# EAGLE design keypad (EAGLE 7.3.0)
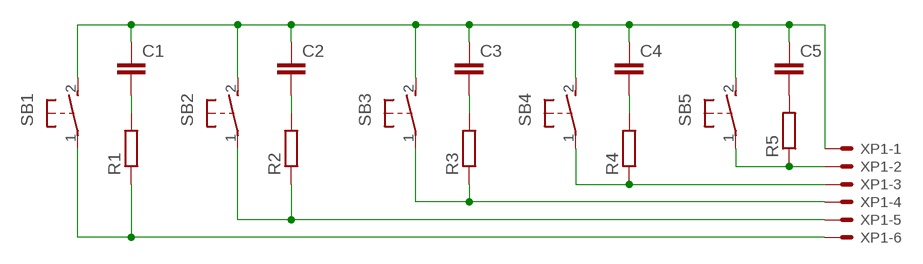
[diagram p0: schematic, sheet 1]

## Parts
C1  C-EUC0603  [C0603]
C2  C-EUC0603  [C0603]
C3  C-EUC0603  [C0603]
C4  C-EUC0603  [C0603]
C5  C-EUC0603  [C0603]
R1  R-EU_R0603  [R0603]
R2  R-EU_R0603  [R0603]
R3  R-EU_R0603  [R0603]
R4  R-EU_R0603  [R0603]
R5  R-EU_R0603  [R0603]
SB1  DTSM-3  [DTSM-3]
SB2  DTSM-3  [DTSM-3]
SB3  DTSM-3  [DTSM-3]
SB4  DTSM-3  [DTSM-3]
SB5  DTSM-3  [DTSM-3]
XP1  53398-06  [53398-06]

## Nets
COM: C1.1 C2.1 C3.1 C4.1 C5.1 SB1.2 SB2.2 SB3.2 SB4.2 SB5.2 XP1.1
DN: R4.1 SB4.1 XP1.3
ENT: R5.1 SB5.1 XP1.2
MODE: R2.1 SB2.1 XP1.5
N$1: C1.2 R1.2
N$2: C2.2 R2.2
N$3: C3.2 R3.2
N$4: C4.2 R4.2
N$5: C5.2 R5.2
ON: R1.1 SB1.1 XP1.6
UP: R3.1 SB3.1 XP1.4

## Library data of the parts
C1-C5 = resistor:C-EU: CAPACITOR, European symbol
R1-R5 = resistor:R-EU_: RESISTOR, European symbol
SB1-SB5 = switch-tact:DTSM-3
XP1 = con-molex:53?-06: CONNECTOR wire to board 1.25 mm (.049 inch) pitch header; OC_FARNELL: 1125368; OC_NEWARK: unknown

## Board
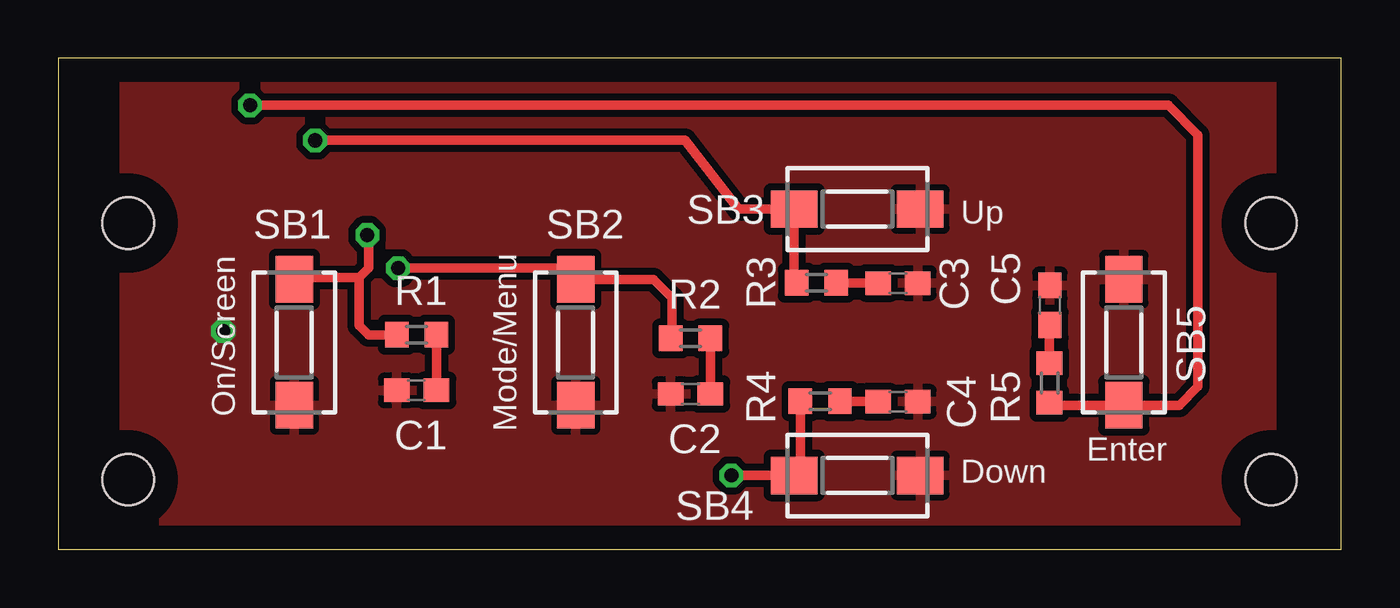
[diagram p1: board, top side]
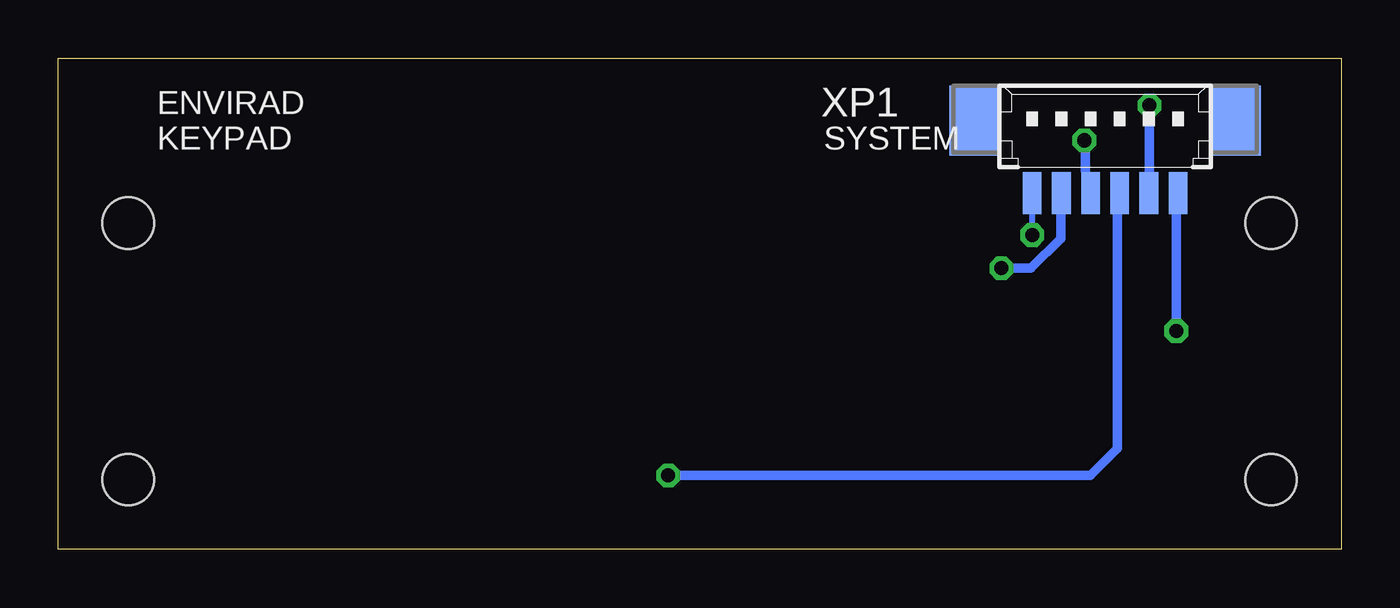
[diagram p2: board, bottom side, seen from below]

Size 55 x 21.07 mm. Coordinates in mm from the lower left corner, seen from the top.
Outline: 0,0 55,0 55,21.07 0,21.07 0,0
Copper layers (1*16): Top 0.035mm / dielectric 1.5mm / Bottom 0.035mm
Design rules "default *": minimum track width 10mil, minimum drill 20mil, track to track 8mil, track to pad 8mil, pad to pad 8mil, via to via 8mil, smd to smd 8mil, copper to edge 40mil, drill to drill 8mil, minimum pad ring 10mil, minimum via ring 8mil, stop-mask expansion 4mil, vias tented up to drill 24mil, thermal gap 10mil
Holes 2.2 mm at 3,3 52,3 52,14 3,14

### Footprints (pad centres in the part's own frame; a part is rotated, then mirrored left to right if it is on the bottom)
C0603 = smd 1.1 x 1: 1 -0.85,0; 2 0.85,0
R0603 = smd 1 x 1.1: 1 -0.85,0; 2 0.85,0
DTSM-3 = smd 2 x 1.6: 1 -2.7,0; 2 2.7,0
53398-06 = smd 0.8 x 1.8: 1 3.125,-2.5; 2 1.875,-2.5; 3 0.625,-2.5; 4 -0.625,-2.5; 5 -1.875,-2.5; 6 -3.125,-2.5 | smd 2.1 x 3: S1 5.625,0.625; S2 -5.625,0.625

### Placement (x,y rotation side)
C1  15.36,6.83 0 top
C2  27.11,6.67 0 top
C3  36,11.43 180 top
C4  36,6.34 180 top
C5  42.51,10.48 270 top
R1  15.36,9.21 0 top
R2  27.11,9.06 0 top
R3  32.5,11.44 0 top
R4  32.66,6.36 0 top
R5  42.49,7.14 90 top
SB1  10.12,8.89 270 top
SB2  22.18,8.89 270 top
SB3  34.25,14.61 0 top
SB4  34.25,3.17 0 top
SB5  45.68,8.89 90 top
XP1  10.12,17.78 0 bottom

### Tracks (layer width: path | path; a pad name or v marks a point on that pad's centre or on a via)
COM  (via drill 0.61)
  Top 0.406: 6.95,9.25 v7.07,9.37
  Bottom 0.254: 7.07,15.09 XP1.1
  Bottom 0.406: v7.07,9.37 7.07,15.09
  pour Top (isolate 0.305): 2.82,20.64 52.03,20.64 52.03,0.32 2.82,0.32
DN  (via drill 0.6)
  Top 0.406: v28.85,3.17 SB4.1 31.81,3.44 R4.1
  Bottom 0.254: 9.59,14.63 9.59,15.09 XP1.3
  Bottom 0.406: 9.59,14.63 9.59,4.34 10.76,3.17 v28.85,3.17
ENT  (via drill 0.6)
  Top 0.406: v8.21,19.05 47.59,19.05 48.85,17.78 48.85,6.99 48.06,6.19 SB5.1 42.59,6.19 R5.1
  Bottom 0.406: v8.21,19.05 8.21,15.88 XP1.2
MODE  (via drill 0.6)
  Top 0.406: v14.56,12.06 21.55,12.06 SB2.1 25.52,11.59 26.31,10.79 26.31,9.12 R2.1
  Bottom 0.406: v14.56,12.06 13.29,12.06 12.03,13.34 12.03,15.24 XP1.5
N$1
  Top 0.406: R1.2 C1.2
N$2
  Top 0.406: R2.2 C2.2
N$3
  Top 0.406: R3.2 35.13,11.44 C3.2
N$4
  Top 0.406: R4.2 35.13,6.36 C4.2
N$5
  Top 0.406: R5.2 42.49,9.61 C5.2
ON  (via drill 0.61)
  Top 0.254: 10.27,11.66 SB1.1
  Top 0.406: 10.27,11.66 12.89,11.66 | 12.89,11.66 13.29,12.06 13.29,13.44 v13.24,13.49 | 12.89,11.66 12.89,9.61 13.29,9.21 R1.1
  Bottom 0.254: v13.24,13.49 13.24,15.09 XP1.6
UP  (via drill 0.61)
  Top 0.254: 31.53,14.68 SB3.1
  Top 0.406: v11.01,17.55 26.86,17.55 29.17,14.61 SB3.1 31.55,11.54 R3.1
  Bottom 0.254: 10.96,16.23 10.96,15.32 XP1.4
  Bottom 0.406: 10.96,16.23 10.96,17.5 v11.01,17.55

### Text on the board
tNames: Up | On/Screen | Mode/Menu | Enter | Down
bNames: SYSTEM | ENVIRAD / KEYPAD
